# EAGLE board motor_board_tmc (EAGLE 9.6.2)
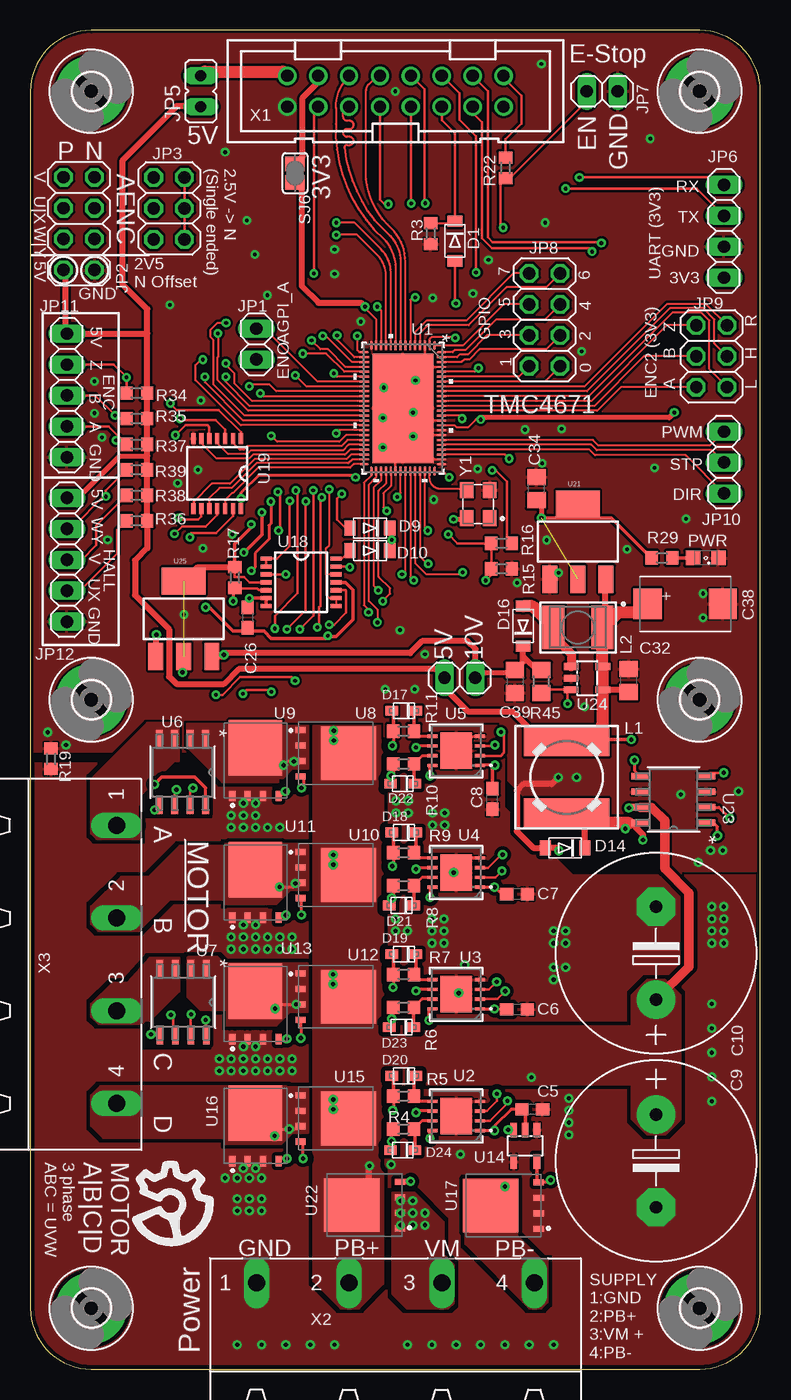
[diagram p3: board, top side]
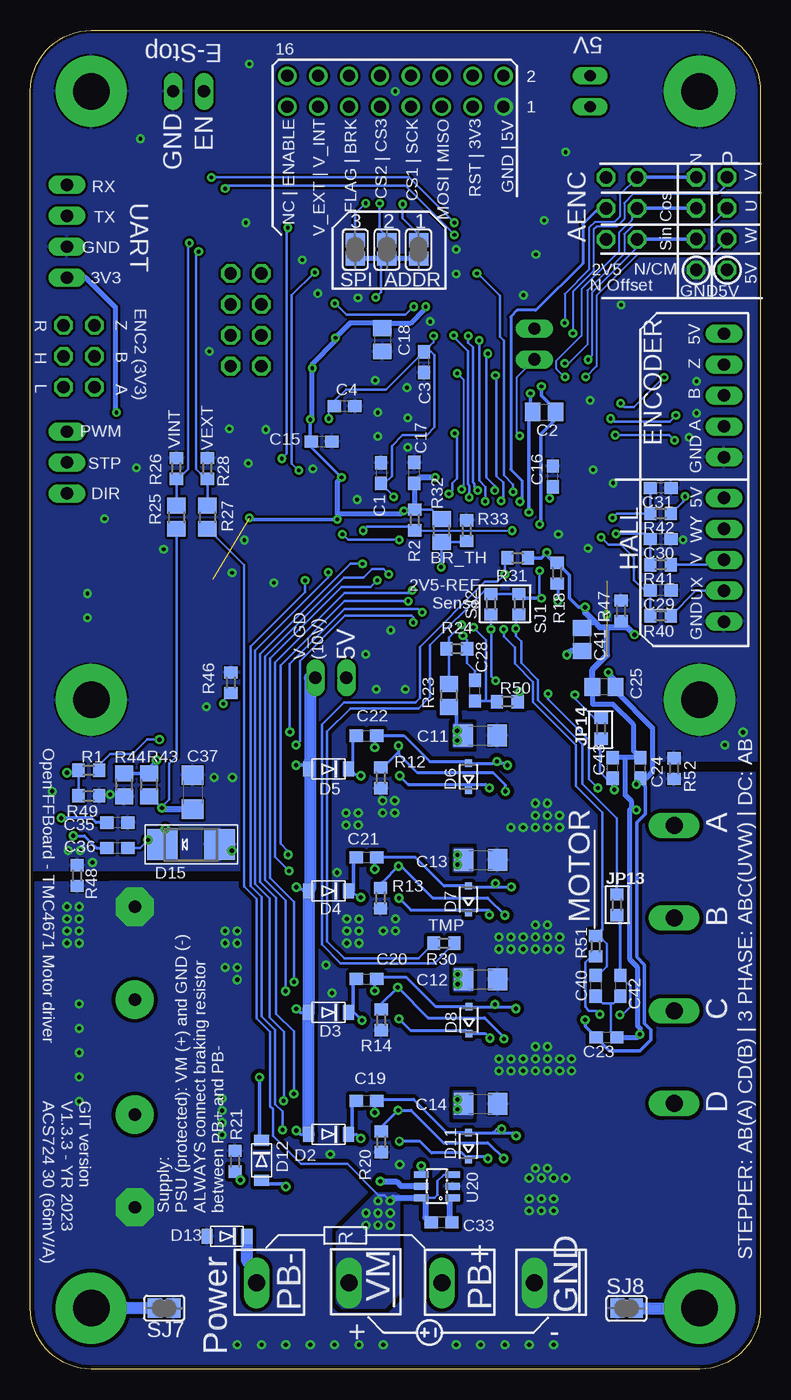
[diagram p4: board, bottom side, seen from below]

Size 60 x 110 mm. Coordinates in mm from the lower left corner, seen from the top.
Outline: 0,5 arc90 5,0 55,0 arc90 60,5 60,105 arc90 55,110 5,110 arc90 0,105 0,5
Copper layers (1*16): Top 0.07mm / dielectric 1.5mm / Bottom 0.07mm
Design rules "jlcpcb *": minimum track width 5mil, minimum drill 0.3mm, track to track 8mil, track to pad 8mil, pad to pad 8mil, via to via 8mil, smd to smd 5mil, copper to edge 0.2mm, drill to drill 8mil, minimum pad ring 10mil, minimum via ring 8mil, stop-mask expansion 4mil, vias tented up to drill 0.4mm, thermal gap 6mil

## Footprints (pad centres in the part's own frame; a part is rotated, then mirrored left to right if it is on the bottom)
C0603 = smd 1.1 x 1: 1 -0.85,0; 2 0.85,0
C0805 = smd 1.3 x 1.5: 1 -0.95,0; 2 0.95,0
E7,5-16 = drill 1.016 pad 3.15: + -3.81,0 | drill 1.016 pad 3.15 octagon: - 3.81,0
C1206 = smd 1.6 x 1.8: 1 -1.4,0; 2 1.4,0
CAPPM7343X310N = smd 2.31 x 2.52: 1 -3.1,0; 2 3.1,0
SOD-123FL = smd 0.91 x 1.22: A 1.637,0; C -1.637,0
SOD323-R = smd 0.6 x 0.6: A 1.1,0; C -1.1,0
SMADIODE = smd 2.54 x 2.54: A 2.349,0; C -2.349,0
SOD-323F = smd 1 x 0.8: A -1,0; C 1,0
3,0-PAD = drill 3 pad 5.842: B3,0 0,0
1X02 = drill 1.016 long: 1 -1.27,0; 2 1.27,0
2X04 = drill 1.016 octagon: 1 -3.81,-1.27; 2 -3.81,1.27; 3 -1.27,-1.27; 4 -1.27,1.27; 5 1.27,-1.27; 6 1.27,1.27; 7 3.81,-1.27; 8 3.81,1.27
2X03 = drill 1.016 octagon: 1 -2.54,-1.27; 2 -2.54,1.27; 3 0,-1.27; 4 0,1.27; 5 2.54,-1.27; 6 2.54,1.27
JP1 = drill 0.914 long: 1 0,-1.27; 2 0,1.27
1X04 = drill 1.016 long: 1 -3.81,0; 2 -1.27,0; 3 1.27,0; 4 3.81,0
1X03 = drill 1.016 long: 1 -2.54,0; 2 0,0; 3 2.54,0
1X05 = drill 1.016 long: 1 -5.08,0; 2 -2.54,0; 3 0,0; 4 2.54,0; 5 5.08,0
RESISTOR_R0603 = smd 1 x 1.1: 1 -0.85,0; 2 0.85,0
8MMINDUCTOR = smd 2.5 x 7: 1 -3,0; 2 3,0
L4532P = smd 1.8 x 3.6: 1 -2,0; 2 2,0
SML0805 = smd 1.2 x 1.2: A 1.05,0; C -1.05,0
R0603 = smd 1 x 1.1: 1 -0.85,0; 2 0.85,0
R0805 = smd 1.3 x 1.5: 1 -0.95,0; 2 0.95,0
SJ = smd 1.168 x 1.6: 1 -0.762,0; 2 0.762,0
QFN76_10P5X6P5 = smd 0.152 x 0.755: 1 -2.6,-5.173; 2 -2.2,-5.173; 3 -1.8,-5.173; 4 -1.4,-5.173; 5 -1,-5.173; 6 -0.6,-5.173; 7 -0.2,-5.173; 8 0.2,-5.173; 9 0.6,-5.173; 10 1,-5.173; 11 1.4,-5.173; 12 1.8,-5.173; 13 2.2,-5.173; 14 2.6,-5.173; 39 2.6,5.173; 40 2.2,5.173; 41 1.8,5.173; 42 1.4,5.173; 43 1,5.173; 44 0.6,5.173; 45 0.2,5.173; 46 -0.2,5.173; 47 -0.6,5.173; 48 -1,5.173; 49 -1.4,5.173; 50 -1.8,5.173; 51 -2.2,5.173; 52 -2.6,5.173 | smd 0.755 x 0.152: 15 3.179,-4.6; 16 3.179,-4.2; 17 3.179,-3.8; 18 3.179,-3.4; 19 3.179,-3; 20 3.179,-2.6; 21 3.179,-2.2; 22 3.179,-1.8; 23 3.179,-1.4; 24 3.179,-1; 25 3.179,-0.6; 26 3.179,-0.2; 27 3.179,0.2; 28 3.179,0.6; 29 3.179,1; 30 3.179,1.4; 31 3.179,1.8; 32 3.179,2.2; 33 3.179,2.6; 34 3.179,3; 35 3.179,3.4; 36 3.179,3.8; 37 3.179,4.2; 38 3.179,4.6; 53 -3.179,4.6; 54 -3.179,4.2; 55 -3.179,3.8; 56 -3.179,3.4; 57 -3.179,3; 58 -3.179,2.6; 59 -3.179,2.2; 60 -3.179,1.8; 61 -3.179,1.4; 62 -3.179,1; 63 -3.179,0.6; 64 -3.179,0.2; 65 -3.179,-0.2; 66 -3.179,-0.6; 67 -3.179,-1; 68 -3.179,-1.4; 69 -3.179,-1.8; 70 -3.179,-2.2; 71 -3.179,-2.6; 72 -3.179,-3; 73 -3.179,-3.4; 74 -3.179,-3.8; 75 -3.179,-4.2; 76 -3.179,-4.6 | smd 5.004 x 8.992: 77 0,0
SDC08A = smd 0.254 x 0.813: 1 -1.2,-1.943; 2 -0.4,-1.943; 3 0.4,-1.943; 4 1.2,-1.943; 5 1.2,1.943; 6 0.4,1.943; 7 -0.4,1.943; 8 -1.2,1.943 | smd 2.997 x 2.591: 9 0,0
SOIC8_D_TEX = smd 1.46 x 0.559: 1 -2.724,1.905; 2 -2.724,0.635; 3 -2.724,-0.635; 4 -2.724,-1.905; 5 2.724,-1.905; 6 2.724,-0.635; 7 2.724,0.635; 8 2.724,1.905
MOSFET_BSC093N04LSGATMA1 = smd 0.5 x 0.85: 1 -1.905,-2.9; 2 -0.635,-2.9; 3 0.635,-2.9; 4 1.905,-2.9 | smd 4.41 x 4.55: 5 0,1.05
SOT23-5L = smd 0.55 x 1.2: 1 -0.95,-1.3; 2 0,-1.3; 3 0.95,-1.3; 4 0.95,1.3; 5 -0.95,1.3
TSSOP14 = smd 0.9 x 0.35: 1 -2.875,1.95; 2 -2.875,1.3; 3 -2.875,0.65; 4 -2.875,0; 5 -2.875,-0.65; 6 -2.875,-1.3; 7 -2.875,-1.95; 8 2.875,-1.95; 9 2.875,-1.3; 10 2.875,-0.65; 11 2.875,0; 12 2.875,0.65; 13 2.875,1.3; 14 2.875,1.95
SOT23-6 = smd 0.55 x 1.2: 1 -0.95,-1.3; 2 0,-1.3; 3 0.95,-1.3; 4 0.95,1.3; 5 0,1.3; 6 -0.95,1.3
SOT223 = smd 1.219 x 2.235: 1 -2.311,-3.099; 2 0,-3.099; 3 2.311,-3.099 | smd 3.6 x 2.2: 4 0,3.099
21-0041B_8_MXM = smd 0.543 x 1.455: 1 -1.905,-2.721; 2 -0.635,-2.721; 3 0.635,-2.721; 4 1.905,-2.721; 5 1.905,2.721; 6 0.635,2.721; 7 -0.635,2.721; 8 -1.905,2.721
PAK100/2500-16 = drill 1 pad 1.422: 1 -8.89,-1.27; 2 -8.89,1.27; 3 -6.35,-1.27; 4 -6.35,1.27; 5 -3.81,-1.27; 6 -3.81,1.27; 7 -1.27,-1.27; 8 -1.27,1.27; 9 1.27,-1.27; 10 1.27,1.27; 11 3.81,-1.27; 12 3.81,1.27; 13 6.35,-1.27; 14 6.35,1.27; 15 8.89,-1.27; 16 8.89,1.27
GMSTBA4 = drill 1.397 long: 1 -11.43,5.08; 2 -3.81,5.08; 3 3.81,5.08; 4 11.43,5.08
ECS-327KE-TR = smd 1.3 x 1.1: 1 -1.15,-0.95; 2 1.15,-0.95; 3 1.15,0.95; 4 -1.15,0.95

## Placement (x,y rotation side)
C1  100nF  [C0603]  31.18,73.62 270 bottom
C2  10µF  [C0805]  17.77,78.65 0 bottom
C3  100nF  [C0603]  27.65,82.75 90 bottom
C4  100nF  [C0603]  34.17,79.12 180 bottom
C5  100nF  [C0603]  41.25,21.35 180 top
C6  100nF  [C0603]  40,29.55 180 top
C7  100nF  [C0603]  40,39.03 180 top
C8  100nF  [C0603]  37.98,46.85 90 top
C9  680µF  [E7,5-16]  51.42,17.1 270 top
C10  680µF  [E7,5-16]  51.42,34.17 90 top
C11  1µF  [C1206]  23.02,52.05 0 bottom
C12  1µF  [C1206]  22.98,32.03 0 bottom
C13  1µF  [C1206]  23,41.85 0 bottom
C14  1µF  [C1206]  23,21.8 0 bottom
C15  100nF  [C0603]  36.08,76.22 0 bottom
C16  100nF  [C0603]  17.05,73.35 90 bottom
C17  100nF  [C0603]  28.45,73.65 90 bottom
C18  10µF  [C0805]  31.07,84.58 270 bottom
C19  100nF  [C0603]  32.38,22.05 0 bottom
C20  100nF  [C0603]  32.38,32.05 0 bottom
C21  100nF  [C0603]  32.38,42.05 0 bottom
C22  100nF  [C0603]  32.38,52.05 0 bottom
C23  100nF  [C0603]  12.65,27.25 180 bottom
C24  100nF  [C0603]  9.88,49.4 90 bottom
C25  10µF  [C0805]  12.85,56.05 180 bottom
C26  100nF  [C0603]  17.85,61.75 270 top
C28  4.7nF  [C0603]  23.45,55.75 90 bottom
C29  4.7nF  [C0603]  8.2,64 180 bottom
C30  4.7nF  [C0603]  8.2,68.2 180 bottom
C31  4.7nF  [C0603]  8.2,72.4 180 bottom
C32  10µF  [C0805]  49.17,56.58 90 top
C33  100nF  [C0603]  26.2,12.05 180 bottom
C34  10µF  [C0805]  41.6,72.35 90 top
C35  100nF  [C0603]  52.85,44.9 180 bottom
C36  100nF  [C0603]  52.85,42.83 0 bottom
C37  1µF  [C1206]  46.67,47.4 270 bottom
C38  593D476X0016D2TE3  [CAPPM7343X310N]  53.83,62.88 0 top
C39  10µF  [C0805]  39.83,56.5 270 top
C40  4.7nF  [C0603]  13.55,31.5 270 bottom
C41  10µF  [C0805]  14.65,59.95 90 bottom
C42  100nF  [C0603]  11.5,31.5 270 bottom
C43  100nF  [C0603]  12.15,49.4 90 bottom
D1  LV low drop  [SOD-123FL]  34.9,92.7 270 top
D2  HV >100V  [SOD-123FL]  35.5,19.3 180 bottom
D3  HV >100V  [SOD-123FL]  35.5,29.3 180 bottom
D4  HV >100V  [SOD-123FL]  35.5,39.3 180 bottom
D5  HV >100V  [SOD-123FL]  35.5,49.3 180 bottom
D6  BZX384-XXX  [SOD323-R]  24,48.67 90 bottom
D7  BZX384-XXX  [SOD323-R]  24,38.6 90 bottom
D8  BZX384-XXX  [SOD323-R]  23.95,28.67 90 bottom
D9  LV low drop  [SOD-123FL]  27.9,69.1 180 top
D10  LV low drop  [SOD-123FL]  27.9,67.25 180 top
D11  BZX384-XXX  [SOD323-R]  24,18.33 90 bottom
D12  HV >100V  [SOD-123FL]  41,17.15 270 bottom
D13  Zener 65V (MMSZ5265BT1G)  [SOD-123FL]  43.85,10.9 180 bottom
D14  HV >100V  [SOD-123FL]  43.95,42.83 180 top
D15  HV >100V  [SMADIODE]  46.8,43.1 0 bottom
D16  LV low drop  [SOD-123FL]  40.5,61.05 90 top
D17  [SOD-323F]  30.7,54.1 0 top
D18  [SOD-323F]  30.7,44.1 0 top
D19  [SOD-323F]  30.7,34.1 0 top
D20  [SOD-323F]  30.7,24.1 0 top
D21  [SOD-323F]  30.5,38.1 0 top
D22  [SOD-323F]  30.6,48.1 0 top
D23  [SOD-323F]  30.5,28.1 0 top
D24  [SOD-323F]  30.6,18 0 top
H1  MOUNT-PAD-ROUND3.0  [3,0-PAD]  55,5 0 top
H2  MOUNT-PAD-ROUND3.0  [3,0-PAD]  5,5 0 top
H3  MOUNT-PAD-ROUND3.0  [3,0-PAD]  55,105 0 top
H4  MOUNT-PAD-ROUND3.0  [3,0-PAD]  55,55 0 top
H5  MOUNT-PAD-ROUND3.0  [3,0-PAD]  5,105 0 top
H6  MOUNT-PAD-ROUND3.0  [3,0-PAD]  5,55 0 top
JP1  [1X02]  18.57,84.22 90 top
JP2  [2X04]  4,94.12 90 top
JP3  [2X03]  11.4,95.38 270 top
JP4  V_DRV  [1X02]  35.3,56.8 180 top
JP5  [JP1]  14,105 0 top
JP6  [1X04]  57,93.5 270 top
JP7  [1X02]  47,105 180 top
JP8  [2X04]  42.27,86.22 90 top
JP9  [2X03]  56,83.22 90 top
JP10  [1X03]  57,74.5 270 top
JP11  [1X05]  3,80 270 top
JP12  [1X05]  3,66.5 270 top
JP13  JUMPER-SMT_2_NO_SILK  [RESISTOR_R0603]  11.8,38.15 90 bottom
JP14  JUMPER-SMT_2_NO_SILK  [RESISTOR_R0603]  13.1,52.65 90 bottom
L1  220µH  [8MMINDUCTOR]  44.08,48.62 90 top
L2  10µH  [L4532P]  45,60.95 180 top
LED1  Green  [SML0805]  55.5,66.65 180 top
R1  47k  [R0603]  55.2,49.2 0 bottom
R2  10k  [R0603]  28.4,69.78 90 bottom
R3  10k  [R0603]  32.9,93.3 90 top
R4  10  [R0603]  30.68,19.72 0 top
R5  10  [R0603]  30.68,22.42 0 top
R6  10  [R0603]  30.68,29.72 0 top
R7  10  [R0603]  30.68,32.42 0 top
R8  10  [R0603]  30.68,39.72 0 top
R9  10  [R0603]  30.68,42.42 0 top
R10  10  [R0603]  30.68,49.73 0 top
R11  10  [R0603]  30.68,52.42 0 top
R12  36k  [R0603]  31.2,48.58 90 bottom
R13  36k  [R0603]  31.23,38.7 90 bottom
R14  36k  [R0603]  31.18,28.7 90 bottom
R15  10k  [R0603]  38.73,65.75 180 top
R16  1.5k  [R0603]  38.73,67.85 180 top
R17  10k  [R0603]  16.8,65.05 90 top
R18  10k  [R0603]  16.7,65.4 270 bottom
R19  0  [R0603]  1.7,50.15 270 top
R20  36k  [R0603]  31.15,18.67 90 bottom
R21  36k  [R0603]  43.17,17.08 270 bottom
R22  1.5k  [R0603]  39.05,98.7 90 top
R23  71.5k  [R0805]  25.6,55.35 270 bottom
R24  1.5k  [R0603]  24.95,59.2 180 bottom
R25  294k  [R0805]  48,70 270 bottom
R26  10k  [R0603]  48,74 270 bottom
R27  294k  [R0805]  45.45,70 270 bottom
R28  10k  [R0603]  45.45,74 270 bottom
R29  1.5k  [R0603]  51.9,66.65 180 top
R30  10k thermistor  [R0603]  26,35 180 bottom
R31  1.5k  [R0603]  19.95,66.65 180 bottom
R32  71.5k  [R0805]  26.2,68.9 90 bottom
R33  47k  [R0603]  24.15,68.9 270 bottom
R34  4.7k  [R0603]  8.75,80.2 0 top
R35  4.7k  [R0603]  8.75,78.1 0 top
R36  4.7k  [R0603]  8.75,69.7 0 top
R37  4.7k  [R0603]  8.75,76 0 top
R38  4.7k  [R0603]  8.75,71.8 0 top
R39  4.7k  [R0603]  8.75,73.9 0 top
R40  1.5k  [R0603]  8.2,61.9 0 bottom
R41  1.5k  [R0603]  8.2,66.1 0 bottom
R42  1.5k  [R0603]  8.2,70.3 0 bottom
R43  294k  [R0805]  50.25,48 270 bottom
R44  71.5k  [R0805]  52.3,48 270 bottom
R45  71.5k  [R0805]  42,56.5 90 top
R46  10k  [R0603]  43.52,56.4 270 bottom
R47  0  [R0603]  11.45,62.3 90 bottom
R48  0  [R0603]  56.15,40.55 270 bottom
R49  15k  [R0603]  55.2,47.1 180 bottom
R50  1.5k  [R0603]  20.8,54.85 0 bottom
R51  1.5k  [R0603]  13.55,34.75 270 bottom
R52  0  [R0603]  7.1,49.35 270 bottom
SJ1  0R  [RESISTOR_R0603]  22.15,62.85 270 bottom
SJ2  0R  [RESISTOR_R0603]  19.85,62.85 270 bottom
SJ3  [SJ]  28.1,92 270 bottom
SJ4  [SJ]  30.7,92 270 bottom
SJ5  [SJ]  33.3,92 270 bottom
SJ6  3.3V  [SJ]  21.75,98.28 270 top
SJ7  [SJ]  49,5 180 bottom
SJ8  [SJ]  11,5 0 bottom
U1  TMC4671  [QFN76_10P5X6P5]  30.62,78.95 180 top
U2  LM5109BSD  [SDC08A]  35,20.8 90 top
U3  LM5109BSD  [SDC08A]  35,30.8 90 top
U4  LM5109BSD  [SDC08A]  35,40.8 90 top
U5  LM5109BSD  [SDC08A]  35,50.8 90 top
U6  TMCS1100  [SOIC8_D_TEX]  12.5,49.05 270 top
U7  TMCS1100  [SOIC8_D_TEX]  12.55,30.15 270 top
U8  BSC030N08NS5ATMA1  [MOSFET_BSC093N04LSGATMA1]  25.1,50.6 270 top
U9  BSC030N08NS5ATMA1  [MOSFET_BSC093N04LSGATMA1]  18.5,50 0 top
U10  BSC030N08NS5ATMA1  [MOSFET_BSC093N04LSGATMA1]  25.1,40.6 270 top
U11  BSC030N08NS5ATMA1  [MOSFET_BSC093N04LSGATMA1]  18.5,40 0 top
U12  BSC030N08NS5ATMA1  [MOSFET_BSC093N04LSGATMA1]  25.1,30.6 270 top
U13  BSC030N08NS5ATMA1  [MOSFET_BSC093N04LSGATMA1]  18.5,30 0 top
U14  MCP14XX  [SOT23-5L]  40.67,18.35 180 top
U15  BSC030N08NS5ATMA1  [MOSFET_BSC093N04LSGATMA1]  25.1,20.6 270 top
U16  BSC030N08NS5ATMA1  [MOSFET_BSC093N04LSGATMA1]  18.5,20 0 top
U17  BSC030N08NS5ATMA1  [MOSFET_BSC093N04LSGATMA1]  38.88,13.42 90 top
U18  MCP6004  [TSSOP14]  22.25,64.65 0 top
U19  74LV17APWJ  [TSSOP14]  15.35,73.6 270 top
U20  LM74700-Q1  [SOT23-6]  26.57,15.03 90 bottom
U21  [SOT223]  45,68 0 top
U22  BSC030N08NS5ATMA1  [MOSFET_BSC093N04LSGATMA1]  27.48,13.47 90 top
U23  MAX5033BASA+T  [21-0041B_8_MXM]  52.85,46.8 90 top
U24  AP3012KTR-G1  [SOT23-5L]  45.75,56.77 270 top
U25  [SOT223]  12.6,61.65 0 top
X1  2516-  [PAK100/2500-16]  30,105 0 top
X2  GMSTBA4  [GMSTBA4]  30,2 0 top
X3  GMSTBA4  [GMSTBA4]  2,33.25 270 top
Y1  25MHz  [ECS-327KE-TR]  36.8,71.08 90 top

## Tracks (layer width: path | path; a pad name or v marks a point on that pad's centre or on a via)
2.5V_REF  (via drill 0.3)
  Top 0.2: JP3.2 JP3.4 JP3.6
  Top 0.254: v18.15,65.6 18.47,65.92 18.47,67.05 19.62,68.19 19.62,69.33 19.77,69.48 v19.77,71.28
  Top 0.3: C26.1 17.85,63.2 v18,63.35
  Top 0.305: U18.7 U18.6 v18,63.35
  Bottom 0.2: 19.85,63.35 SJ2.1 SJ1.1 22.36,63.91 22.72,63.91 27.15,59.48 27.15,55.25 28.1,54.3 33.7,54.3 35.6,52.4 35.6,35.15 34.2,33.75 28.1,33.75 R30.2 | v18.15,65.6 18.15,63.5 v18,63.35
  Bottom 0.254: JP3.4 12.82,95.53 13.16,95.53 14.61,94.08 14.61,90.85 18.46,87 20,87 20.52,86.48 20.52,73.92 19.62,73.01 19.62,71.43 v19.77,71.28
  Bottom 0.305: 19.85,63.35 v18,63.35
2.5V_REF_A  (via drill 0.3)
  Top 0.152: U1.17 26.44,82.75 24.29,84.9 v24.02,84.9
  Top 0.2: v23.24,72.2 23.29,72.15 23.29,61.94 v22.15,60.8 | v15.25,55.4 15.79,55.4 17.25,56.86 21.45,56.86 v21.75,56.56
  Bottom 0.2: v24.02,84.9 24.02,84.34 23.64,83.96 23.64,72.89 23.49,72.74 23.49,72.46 v23.24,72.2 | SJ1.2 v22.15,60.8 22.09,60.74 22.09,56.9 v21.75,56.56 | v15.25,55.4 15.25,55.1 13.65,53.5 JP14.2
2.5V_REF_C  (via drill 0.3)
  Top 0.152: U1.19 25.8,81.95 24.3,83.44 v22.4,83.44
  Top 0.2: v21.82,72.19 21.97,72.05 21.97,63.77 20.1,61.9 v20.1,60.85
  Bottom 0.2: v22.4,83.44 22.54,83.31 22.54,73.25 21.82,72.54 v21.82,72.19 | SJ2.2 20.1,61.75 v20.1,60.85 20.1,60.25 19.65,59.8 19.65,58 18.27,56.62 18.27,54.98 14.63,51.34 14.63,48.07 11.8,45.24 JP13.2
2.5V_REF_RAW  (via drill 0.35)
  Top 0.2: R17.1 16.85,64.15 18.62,64.15 18.77,64 U18.5
  Top 0.25: R17.1 16.65,64.05 v16.65,63.1
  Bottom 0.25: R18.2 16.65,64.5 v16.65,63.1
5V_SENSE  (via drill 0.3, 0.35)  (1 unrouted)
  Top 0.152: U1.23 20.2,80.35 19.65,80.9 18.15,80.9 v18,80.75
  Top 0.2: U18.4 18.02,64.65 17.57,65.1 16.8,65.1 R17.2 16.7,65.8
  Top 0.254: 14.4,47.75 14.4,47.74 U6.8 | v14.4,28.7 14.46,28.64 U7.8
  Top 0.3: 14.4,47.75 13.5,48.65 10.8,48.65 v10.2,48.05 | 13.25,64.75 U25.4 | R17.2 16.8,67.8 18.14,69.15 v18.14,69.41
  Top 0.5: U25.2 12.5,58.45 v12.5,57.25 | U25.4 13.75,65.9 R17.2
  Bottom 0.2: v18.14,69.41 18.03,69.29 | v10.2,48.05 10.2,48.23 C24.1
  Bottom 0.3: v14.4,28.7 14.4,28.15 C23.2 12.4,26.15 9.9,26.15 9,27.05 9,27.88 9.53,28.41 9.53,33.23 10.17,33.87 10.17,44.92 9.47,45.62 9.47,47.88 9.88,48.29 C24.1 | v18,80.75 18,79.97 16.82,78.8 C2.2 16.82,78.05 18.03,76.85 18.03,69.29
  Bottom 0.4: C24.1 9.43,48.55 8.85,49.12 8.85,52.65 11.9,55.7 C25.1 11.45,56.5
  Bottom 0.5: v12.5,57.25 12.5,57.1 11.9,56.5 C25.1
+3V3  (via drill 0.3)  (1 unrouted)
  Top 0.152: U1.52 33.25,73.75 33.95,73.75 v34.42,73.28 | U1.43 29.62,72.58 29.02,71.98 29.02,70.81 v29.3,70.53 | U1.13 28.42,86.28 27.5,87.19 v27.5,87.3 | v34.92,84.75 34.92,84.8 33,84.8 32.82,84.62 U1.2 | v36.83,82.25 36.52,81.95 U1.72 | v37,78.03 36.6,78.03 35.99,77.42 35,77.42 34.87,77.55 U1.61
  Top 0.2: v17.32,71.56 17.32,70.75 U19.14
  Top 0.254: v26.73,73.28 26.57,73.42 18.74,73.42 17.32,72 v17.32,71.56
  Top 0.3: v42,69.95 45,69.95 | R29.2 47.75,69.95 45,69.95 | U21.4 45,69.95
  Top 0.4: Y1.4 35.75,69.83 v34.77,69.83 | v52.92,78.6 52.5,78.17 37.15,78.17 v37,78.03 | C34.1 42,71 v42,69.95
  Top 0.5: v27.5,87.3 27.18,87.62 23.68,87.62 22.3,89 22.3,96.96 SJ6.2
  Bottom 0.2: v29.3,70.53 29.2,70.62 R2.2 26.98,70.62 R32.2 | C15.1 37,76.3 | v17.32,71.56 17.32,72.23 C16.1
  Bottom 0.254: v34.42,73.28 36.92,75.78 C15.1
  Bottom 0.3: v27.5,87.3 27.6,87.2 | 36.91,78.12 v37,78.03 37,76.3 | v42,69.95 41.88,69.83 v34.77,69.83
  Bottom 0.4: 34.77,70.28 v34.77,69.83 | 27.6,87.2 27.6,87.1 28.77,85.92 31.07,85.92 | 36.91,78.12 36.91,82.17 v36.83,82.25 36.83,82.6 34.92,84.5 v34.92,84.75 33.73,85.95 31.07,85.95 31.07,85.92 | C17.1 28.45,71 28.93,70.53 v29.3,70.53 29.55,70.28 34.77,70.28 | v52.92,78.6 53,78.67 53,87.22 55.47,89.69 JP6.4 | C18.1 31.07,85.92 | 34.77,70.28 34.77,72.92 v34.42,73.28
  Bottom 0.5: v26.73,73.28 27.98,73.28 C17.1
+5V  (via drill 0.35)
  Top 0.2: 47.21,61.16 L2.1
  Top 0.254: C38.1 50.02,62.17 50,62.17
  Top 0.3: v49.4,51.73 46.73,51.73 46.62,51.62
  Top 0.4: JP12.1 3.88,71.58 7.33,75.03 9.6,75.03
  Top 0.5: 9.6,85.1 9.58,85.08 JP11.1 2.88,85.2 2.88,90.17 JP2.2 | 9.6,85.1 R34.2 R35.2 R37.2 9.6,75.03 R39.2 R38.2 R36.2 9.6,67.45 8.6,66.45 8.6,63.6 11.4,60.8 11.4,56.9 12,56.3 15.9,56.3 17.11,57.51 33.32,57.51 JP4.2 34.33,56.5 34.33,55.67 35.95,54.05 39.6,54.05 42.02,51.62 L1.2 45.62,51.62 47,53 | 9.6,85.1 9.6,87.1 7.6,89.1 7.6,99.35 12.03,103.78 13.95,103.78 JP5.1 | 47,55.77 U24.4 48.98,55.83 C32.1 | 47,52 46.62,51.62 | U21.3 47.21,64.8 47.21,61.16
  Top 0.8: U24.5 47,57.77
  Top 1: C38.1 51.26,63.41 | U24.4 U24.5 | 47,55.77 47,53 47,52 | 47,57.77 L2.1 47.1,60.95 48.33,62.17 50,62.17 51,62.17 51,63
  Bottom 0.2: v49.4,51.73 50.4,51.73 51.58,50.55 53.45,50.55 54.2,49.8 54.2,49.35 R1.2
AENC_UX  (via drill 0.3)
  Top 0.15: 18.2,79.55 16.75,81 16.75,81.83 16.07,82.5 v16.07,82.65
  Top 0.152: U1.25 18.2,79.55
  Bottom 0.15: 14.22,88.62 14.22,84.17 15.75,82.65 v16.07,82.65
  Bottom 0.152: 10.41,94.05 11.19,93.27 11.19,91.66 14.22,88.62 | JP2.6 2.73,95.34
  Bottom 0.2: 10.41,94.05 4.02,94.05 2.73,95.34
AENC_UX_N  (via drill 0.3)
  Top 0.15: U1.26 18.02,79.15 16.05,81.12 v16.05,81.53
  Bottom 0.152: v16.05,81.53 16.1,81.53 16.75,82.17 16.75,82.87 14.7,84.92 14.7,88.72 11.61,91.81 11.61,93.39 10.58,94.43 10.58,94.93 JP3.3 10.11,95.39
  Bottom 0.3: JP2.5 10.11,95.39
AENC_VN  (via drill 0.3)
  Top 0.15: U1.27 17.91,78.75
  Top 0.152: 17.91,78.75 15.39,81.27 15.39,83.14 15.41,83.16 v15.41,85.11
  Bottom 0.152: 10.43,96.6 11.2,95.83 11.2,94.47 11.78,93.89 13.46,93.89 13.72,93.62 13.72,90.2 15.41,88.52 v15.41,85.11
  Bottom 0.2: 2.72,97.38 3.5,96.6 10.43,96.6 | JP2.8 2.72,97.92
  Bottom 0.3: 2.72,97.92 2.72,97.38
AENC_VN_N  (via drill 0.3)
  Top 0.15: U1.28 17.62,78.35 15.04,80.94
  Top 0.152: v16.08,85.96 15.36,85.96 14.78,85.37 14.78,84.84 15.04,84.58 15.04,80.94
  Bottom 0.152: v16.08,85.96 16.08,88.35 14.08,90.35 14.08,93.77 13.61,94.25 12.01,94.25 11.56,94.7 11.56,96.49 JP3.1 10.11,97.94
  Bottom 0.3: JP2.7 10.11,97.94
AENC_WY  (via drill 0.3)
  Top 0.15: U1.29 17.48,77.95 14.35,81.08 v14.35,81.53
  Bottom 0.152: 10.03,91.67 13.47,88.22 13.47,82.4 v14.35,81.53 | JP2.4 2.73,92.8
  Bottom 0.2: 10.03,91.67 3.85,91.67 2.73,92.8
AENC_WY_N  (via drill 0.3)
  Top 0.15: U1.30 17.28,77.55 13.57,81.26 13.57,82.5
  Top 0.152: 13.57,82.5 14.03,82.95 v14.17,82.95
  Bottom 0.152: v14.17,82.95 13.83,83.29 13.83,88.47 10.13,92.17 JP3.5 10.11,92.86
  Bottom 0.3: JP2.3 10.11,92.86
AGPI_A
  Top 0.152: U1.21 23.6,81.15 19.25,85.5 JP1.2
AGPI_B  (via drill 0.3)
  Top 0.152: U1.22 22.68,80.75 v21.78,81.65
  Top 0.2: U18.2 U18.1 20.27,66.6 21.32,67.64 v21.32,71.35
  Bottom 0.2: v21.78,81.65 21.68,81.55 21.68,73.4 21.12,72.84 21.12,71.55 v21.32,71.35
BRAKE_CTRL  (via drill 0.3, 0.35)
  Top 0.2: D10.C 29.69,67.4 v29.69,68.15 29.69,69.12 29.56,69.12 D9.C | v34.35,68.6 35.1,67.85 R16.2 R15.2 37.88,65.25 v37.42,64.8
  Top 0.254: U14.3 v39.27,19.65
  Bottom 0.2: v37.42,64.8 37.42,63.85 41.92,59.36 41.92,39.71 41,38.79 41,29 39.88,27.88 39.88,21.77 39.27,21.16 v39.27,19.65 | v34.35,68.6 33.9,68.15 v29.69,68.15
BRAKE_CTRL_EXT  (via drill 0.3)
  Top 0.2: X1.12 35.25,104.83 35.25,102.65 36.6,101.3 36.6,90.15 v36.62,90.12 | R16.1 39.17,68.25 39.17,72.92 38.25,73.85 v37.95,73.85
  Bottom 0.2: v36.62,90.12 38.52,88.23 38.52,74.42 v37.95,73.85
BRAKE_CTRL_TMC  (via drill 0.3)
  Top 0.152: U1.31 25.38,77.15 v25.12,76.9
  Top 0.2: v25.6,71.92 25.2,71.53 25.2,69.8 25.9,69.1 D9.A
  Bottom 0.2: v25.12,76.9 24.95,76.72 24.95,73.17 25.3,72.83 25.3,72.22 v25.6,71.92
BRAKE_GATE  (via drill 0.35)
  Top 0.254: v42.75,15.53 42.55,15.33 U17.4
  Top 0.3: U17.4 41.65,15.45 41.65,17.03 U14.5
  Bottom 0.2: R21.2 42.75,16.22 v42.75,15.53
BRAKE_RES_COMP
  Top 0.152: D10.A 25.61,66.6 U18.14
BRAKE_RES_TH  (via drill 0.3)
  Top 0.2: U18.13 26.2,65.95 v26.25,65.9
  Bottom 0.2: R33.2 24.25,67.95 R32.1 26.2,65.95 v26.25,65.9
C_HS_A  (via drill 0.3, 0.35)
  Top 0.152: U1.39 28.02,73.43 27.42,72.83 27.42,62.77 27.79,62.4 v27.79,62.2
  Top 0.2: U5.2 38.67,50.4 38.92,50.65 38.92,52.1 v38.67,52.35
  Bottom 0.2: v38.67,52.35 38.7,52.38 38.7,57.94 34.2,62.45 28.12,62.45 27.87,62.2 v27.79,62.2
C_HS_B  (via drill 0.3, 0.35)
  Top 0.152: U1.41 28.82,73.03 28.22,72.43 28.22,64.38 v28.6,64
  Top 0.2: U4.2 38.23,40.4 v38.75,40.92
  Bottom 0.2: v38.75,40.92 39.9,42.08 39.9,58.08 34.2,63.77 28.82,63.77 v28.6,64
C_HS_C  (via drill 0.3, 0.35)
  Top 0.152: U1.46 30.8,73.75 30.8,65.55 v30.55,65.3
  Top 0.2: U3.2 38.38,30.4 v39.02,31.05
  Bottom 0.2: v39.02,31.05 39.02,38.53 40.71,40.21 40.71,58.54 34.21,65.03 32.64,65.03 31.92,65.75 31,65.75 v30.55,65.3
C_HS_D  (via drill 0.3, 0.35)
  Top 0.152: v35.52,65.47 35.35,65.3 32.55,65.3 31.62,66.23 U1.48
  Top 0.2: U2.2 37.77,20.4 39.2,21.83 v39.2,22.05
  Bottom 0.2: v39.2,22.05 39.15,22.1 39.15,27.72 40.33,28.9 40.33,38.69 41.51,39.87 41.51,59.06 35.52,65.05 v35.52,65.47
C_LS_A  (via drill 0.3, 0.35)
  Top 0.152: U1.40 28.42,73.28 27.82,72.68 27.82,63.1 28.52,62.4 v28.52,61.35
  Top 0.2: U5.3 38.1,51.2 v38.17,51.27
  Bottom 0.2: v38.17,51.27 37.85,51.6 37.85,58.2 34.12,61.92 28.68,61.92 28.52,61.77 v28.52,61.35
C_LS_B  (via drill 0.3, 0.35)
  Top 0.152: U1.42 29.22,72.78 28.62,72.18 28.62,65.1 29.56,64.16 29.56,63.71 v28.95,63.11
  Top 0.2: U4.3 37.62,41.2 38.7,42.28 v38.83,42.28
  Bottom 0.2: v38.83,42.28 38.83,42.55 39.45,43.17 39.45,57.83 34.17,63.11 v28.95,63.11
C_LS_C  (via drill 0.3, 0.35)
  Top 0.152: U1.47 31.22,65.09 v31.5,64.81
  Top 0.2: U3.3 37.7,31.2 v38.33,31.83
  Bottom 0.2: v38.33,31.83 38.33,38.4 40.3,40.37 40.3,58.37 34.42,64.26 32.05,64.26 v31.5,64.81
C_LS_D  (via drill 0.3, 0.35)
  Top 0.152: U1.49 32,73.76 32,66.75 32.58,66.17 v32.7,66.17
  Top 0.2: v38.35,22.62 38.35,22.03 37.52,21.2 U2.3
  Bottom 0.2: v38.35,22.62 38.35,27.75 39.8,29.2 39.8,38.73 41.11,40.04 41.11,58.77 33.7,66.17 v32.7,66.17
CLK_25M
  Top 0.152: Y1.3 35.75,72.33 33.7,72.33 arc-90 32.82,73.21 U1.51
CS1  (via drill 0.3)
  Top 0.2: X1.7 28.73,96.09 29.1,95.72 v29.4,95.72
  Bottom 0.2: SJ3.1 28.1,93.26 29.4,94.56 v29.4,95.72
CS2  (via drill 0.3)
  Top 0.2: X1.9 31.27,95.81 v31.3,95.78
  Bottom 0.2: v31.3,95.78 31.3,93.68 30.7,93.08 SJ4.1
CS3  (via drill 0.3)
  Top 0.2: X1.10 32.38,105.17 32.38,95.78 32.42,95.78 v32.45,95.8
  Bottom 0.2: SJ5.1 33.3,94.95 v32.45,95.8
CS_TMC  (via drill 0.3)
  Top 0.152: 31.43,88.08 31.22,87.87 U1.6
  Top 0.2: v31.62,88.08 31.43,88.08
  Bottom 0.2: v31.62,88.08 31.2,88.5 31.2,90.74 SJ4.2
  Bottom 0.4: SJ3.2 SJ4.2 SJ5.2
DIR
  Top 0.152: JP10.3 53.86,75.1 46.4,75.1 45.95,75.55 U1.56
ENABLE  (via drill 0.3)
  Top 0.152: 39.02,75.15 U1.55
  Top 0.2: v39.35,74.82 39.02,75.15 | v38.85,93.79 38.62,94.02 38.62,97.42 R22.1 39.4,97.85 45.73,104.18 JP7.2
  Bottom 0.2: v38.85,93.79 38.95,93.69 38.95,75.22 v39.35,74.82
ENC2_A
  Top 0.152: JP9.2 48.53,80.69 46.59,78.75 U1.64
ENC2_B
  Top 0.152: JP9.4 50.43,83.22 46.35,79.15 U1.65
ENC2_Z
  Top 0.152: JP9.6 52.33,85.77 46.12,79.55 U1.66
ENC_A
  Top 0.152: U1.35 26.26,75.55 25.85,75.14 18.29,75.14 17.98,74.83 15.31,74.83 14.05,76.09 U19.6
ENC_A_5V  (via drill 0.3)
  Top 0.152: v7.05,76.33 7.58,76.33 R37.1
  Top 0.2: R37.1 6.44,77.46 JP11.4 | U19.5 14.7,77.41 14.55,77.56 12.77,77.56 11.95,76.75 v11.93,76.75
  Bottom 0.2: v7.05,76.33 7.47,76.75 v11.93,76.75
ENC_B
  Top 0.152: U1.34 26.16,75.95 25.7,75.49 18.1,75.49 17.8,75.19 16.25,75.19 15.35,76.09 U19.4
ENC_B_5V  (via drill 0.3)
  Top 0.2: R35.1 7.22,78.1 v6.95,78.38 5.33,80 JP11.3 | U19.3 16,77.18 15.21,77.97 12.3,77.97 v12.3,78.1
  Bottom 0.2: v6.95,78.38 7.45,77.88 12.07,77.88 v12.3,78.1
ENC_Z
  Top 0.152: U1.33 26.05,76.35 25.55,75.85 17.83,75.85 17.52,75.55 17.2,75.55 16.65,76.09 U19.2
ENC_Z_5V  (via drill 0.3)
  Top 0.2: JP11.2 6.86,82.54 v7.9,81.5 R34.1 | U19.1 17.3,77 15.48,78.82 12.03,78.82 v11.5,79.35
  Bottom 0.2: v11.5,79.35 11.2,79.05 10.4,79.05 7.92,81.53 v7.9,81.5
ENO  (via drill 0.3)
  Top 0.152: U1.32 25.95,76.75 25.41,76.21 20.28,76.21 v19.79,76.7
  Bottom 0.152: JP1.1 20.05,81.48 20.05,76.96 v19.79,76.7
FLAG
  Top 0.152: R3.2 34.85,94.15 34.9,94.2 D1.C
  Top 0.2: X1.11 33.81,102.63 34.9,101.54 D1.C
G_HS_A  (via drill 0.35)
  Top 0.254: v22.27,47.75 22.48,47.75 22.48,48.42 U8.4 | R10.1 29.82,48.92 v29.65,48.75
  Top 0.3: D22.A 29.6,48.7 v29.65,48.75
  Bottom 0.2: D6.C 24,48.05
  Bottom 0.254: v22.27,47.75 22.57,48.05 24,48.05 28.95,48.05 v29.65,48.75
G_HS_B  (via drill 0.35)
  Top 0.254: v22.27,37.33 22.27,38.62 U10.4 | R8.1 29.82,38.83 v29.7,38.7
  Top 0.3: D21.A 29.5,38.5 v29.7,38.7
  Bottom 0.2: D7.C 24,37.72
  Bottom 0.254: 24,37.72 22.27,37.72 v22.27,37.33 | v29.7,38.7 28.73,37.72 24.23,37.72 D7.C
G_HS_C  (via drill 0.35)
  Top 0.254: U12.4 22.2,28.1 22.23,28.08 v22.23,27.2 | v29.7,28.78 29.82,28.9 R6.1
  Top 0.3: D23.A 29.5,28.58 v29.7,28.78
  Bottom 0.254: v22.23,27.2 22.6,27.58 D8.C 24.23,27.85 28.77,27.85 v29.7,28.78
G_HS_D  (via drill 0.35)
  Top 0.254: v22.4,17.3 22.4,18.5 U15.4 | v29.68,18.72 29.68,19.58 R4.1
  Top 0.3: D24.A 29.68,18.08 v29.68,18.72
  Bottom 0.2: D11.C 24,17.47
  Bottom 0.254: 24,17.47 22.45,17.47 22.4,17.42 v22.4,17.3 | D11.C 24.52,17.75 27.02,17.75 28,18.72 v29.68,18.72
G_LS_A  (via drill 0.35)
  Top 0.254: U9.4 20.57,47.1 v20.95,47.48 | R11.1 29.82,51.3 v29.75,51.23
  Top 0.3: D17.A 29.82,53.98 R11.1
  Bottom 0.152: R12.2 31.02,49.42 30.73,49.73
  Bottom 0.254: v20.95,47.48 20.95,47.98 21.97,49.01 28.21,49.01 29.75,50.55 | v29.75,51.23 29.75,50.55 | 29.75,50.55 29.82,50.62 30.73,49.73
G_LS_B  (via drill 0.35)
  Top 0.254: U11.4 20.8,37.1 v21,37.3 | R9.1 29.82,41.4 v29.75,41.33
  Top 0.3: D18.A 29.82,43.97 R9.1
  Bottom 0.152: R13.2 31.04,39.74 31.04,40.04
  Bottom 0.254: v21,37.3 22.43,38.72 26.95,38.72 29.55,41.33 v29.75,41.33 31.04,40.04
G_LS_C  (via drill 0.35)
  Top 0.254: U13.4 20.43,27.12 v21.07,27.12 | R7.1 29.82,31.39 v29.8,31.37
  Top 0.3: D19.A 29.82,33.97 R7.1
  Bottom 0.152: R14.2 31.18,29.99
  Bottom 0.254: v21.07,27.12 21.07,27.28 22.68,28.88 27.31,28.88 v29.8,31.37 31.18,29.99
G_LS_D  (via drill 0.35)
  Top 0.254: v21.1,17.3 20.61,17.3 U16.4 | R5.1 29.82,21.32 v29.77,21.27
  Top 0.3: D20.A 29.82,23.97 R5.1
  Bottom 0.152: R20.2 31.15,19.89
  Bottom 0.254: v21.1,17.3 22.4,18.6 26.05,18.6 28.72,21.27 v29.77,21.27 31.15,19.89
GND  (via drill 0.3, 0.35)
  Top 0.152: 30.62,80 30.62,81.87 31.1,82.35 32.5,82.35 | 30.62,80 U1.77 | 30.62,80 30.57,79.95 29,79.95 30,78.95 U1.77 | U1.54 33.25,74.75 31.5,76.5 | 31.42,76.75 31.59,76.59 31.5,76.5 | 31.42,76.75 30.62,77.55 30.62,78 | 30.62,78 U1.77 | U1.62 32.55,77.95 32.5,78 30.62,78 | U1.73 32.5,82.35 | U1.3 32.42,82.43 32.5,82.35 | U1.44 30.02,74.98 30,75 31.5,76.5 | U1.59 31.42,76.75
  Top 0.5: v43.4,48.62 42.85,48.08 40.54,48.08 39.97,47.51 39.97,44.19 41.33,42.83 D14.A 43.23,42.83 v43.45,42.6
  other vias: 16,100 30,105 25,92 36.38,88.38 42.3,94.2 42,107.25 25,90 29.05,80.65 50.95,101.1 11.45,87.45 36.77,73.97 51.3,74.05 17.77,94.4 13.75,73.9 45.3,83.62 31.65,81.25 28.98,78.17 31.45,78.6 28.98,75.75 31.45,76.65 33.15,71.45 27.15,86.08 5.25,81.15 5.25,78.55 6.35,68.15 5.88,76.58 18.45,91.6 12.1,72.8 19.48,88.25 14.18,67.45 37.65,91.15 49.05,67.35 45.55,54.42 40,64.6 43.65,77.25 40.65,77.2 16.6,68.6 44.9,48.62 53.9,69.88 55.3,63.73 14,79.6 30.38,60.73 12.62,62 33.08,88.03 53.45,47.23 55.9,42.62 54.9,41.62 56.9,42.62 1.43,52.33 2.92,51.27 43.42,65.42 42.08,74.42 55.3,61.73 58.2,47.48 29.18,55.88 31.57,55.88 42.42,68.12 32.42,58.73
  pour Bottom (rank 6): -0.45,50 -0.45,111 60.3,111 60.3,41 42.2,41 42.2,50
  pour Top (rank 6): -0.6,50.67 -0.6,111 60.3,111 60.3,40.25 47.35,40.25 36.9,50.7
  pour Top (no thermals): 22,105 20,105 20,102.65 22,102.65
  pour Bottom (no thermals): 22,105 20,105 20,102.65 22,102.65
  cutout Top: 9,45.35 14.85,45.35 14.85,48.5 11.25,48.5 9,46.25
GND1
  cutout Top: 9.2,26.35 14.75,26.35 14.75,28.45 9.5,28.45 9.2,28.15
GNDA  (via drill 0.3, 0.35)
  Top 0.152: v18.9,80.18 19.13,79.95 U1.24
  Top 0.3: U18.11 25.89,64.65 26.53,64.01 26.53,61.59 25.13,60.19 24.5,60.19 v24.45,60.24 24.26,60.05 19.78,60.05 19.2,60.63 18,60.63 | v17.55,67.1 19.02,68.58 v19.02,70.4 | 18,60.63 16.67,60.63 14.7,62.6 v14.4,62.6 | C26.2 18,60.75 18,60.63
  Top 0.4: U7.5 10.57,27.5 v9.9,27.5 | U6.5 10.58,46.33 v10.2,45.95
  Top 0.5: v10.35,60.35 10.29,60.29 U25.1
  Bottom 0.2: 12.3,30.05 12.1,30.05 C42.2 | 12.3,30.05 12.95,30.05 C40.2 | C23.1 12.3,27.75 12.3,30.05 | C28.2 23.45,57.35 24.1,58 R24.1 24.1,59.89 v24.45,60.24
  Bottom 0.25: 23.4,56.65 C28.2
  Bottom 0.3: v18.9,80.18 18.9,78.65 C2.1 19.02,78.35 v19.02,70.4 | 10.72,46 10.57,46 10.25,46 v10.2,45.95 | R31.1 18,66.65 v17.55,67.1 17.55,66.85 16.94,66.24 16.94,66.25 R18.1 15.7,65.25 15.7,63.35 14.95,62.6 v14.4,62.6
  Bottom 0.4: C23.1 10.15,27.25 v9.9,27.5 9.9,28 10.08,28.18 10.08,33 10.72,33.64 10.72,46 | 11.11,50.25 11.11,47.16 10.57,46.62 10.57,46 | 11.11,50.25 C43.2 | 11.11,50.25 C24.2 10.41,50.79 10.41,52.91 12.15,54.65 13.8,54.65 C25.2
  Bottom 0.5: v10.35,60.35 10.95,60.95 11,60.95 | 11,60.95 12.6,60.95 | 12.6,60.95 13.2,60.95 13.62,61.38 | 13.62,61.38 14.4,62.15 v14.4,62.6 | C25.2 13.8,57.48 12.6,58.68 12.6,60.95 | R47.1 11.45,61.4 11,60.95 | C41.2 14.18,61.38 13.62,61.38
GNDI  (via drill 0.35)
  Top 0.2: U3.9 35,30.84 | U4.9 35,41.28 35.36,41.64 | U5.4 35.78,52 35,51.22 U5.9
  Top 0.3: U4.4 35.73,42 35.36,41.64
  other vias: 18.5,45.5 17.5,45.5 16.5,45.5 16.5,44.5 17.5,44.5 19.5,44.5 18.5,44.5 17.5,46.5 20.5,44.5 18.5,46.5 19.5,35.5 18.5,35.5 17.5,35.5 16.5,35.5 16.5,34.5 17.5,34.5 19.5,34.5 18.5,34.5 17.5,36.5 18.5,36.5 20.5,34.5 20.5,35.5 21.5,35.5 21.5,34.5 19.5,25.5 18.5,25.5 17.5,25.5 16.5,25.5 16.5,24.5 17.5,24.5 19.5,24.5 18.5,24.5 15.53,24.5 17.5,26.5 18.5,26.5 15.53,25.5 20.5,24.5 20.5,25.5 21.5,25.5 21.5,24.5 19,13 17,13 19,15.7 18,15.7 17,15.7 16,15.7 17.5,16.5 18.5,16.5 19,14 17,14 18,14 18,13 25,2 23,2 21,2 19,2 17,2 41,2 39,2 37,2 35,2 33,2 31,2 43,2 34.05,44.7 33.05,45.7 34.05,45.7 33.05,44.7 30.05,46.7 31.05,46.7 31.05,45.7 30.05,45.7 34,35 34,36 33,37 30,37 34,37 33,35 33,36 30,36 31,36 35.35,17.65 29.65,16.8 44,36 44,35 44,33 43,32 43,33 43,35 43,36 44.25,19.25 44.25,20.25 44.25,21.25 44.25,22.25 56,36 57,36 57,35 56,35 56,38 57,38 57,37 56,37 56,30 56,28 56,26 56,24 56,22 35.7,33.2 35.2,30.9 34.8,40.8
  pour Top (no thermals): 16.15,44.5 19.5,44.5 19.5,47.7 16.15,47.7
  pour Top (no thermals): 16.15,34.5 19.5,34.5 19.5,37.8 16.15,37.8
  pour Top (no thermals): 16.15,24.5 19.5,24.5 19.5,27.7 16.15,27.7
  pour Top (no thermals): 16.15,15.5 19.5,15.5 19.5,17.7 16.15,17.7
  pour Top (no thermals): 53.42,15.1 49.42,15.1 49.42,11.1 53.42,11.1
  pour Bottom (no thermals): 53.42,15.1 49.42,15.1 49.42,11.1 53.42,11.1
  pour Bottom (no thermals): 53.45,40.03 49.45,40.03 49.45,36.03 53.45,36.03
  pour Top (isolate 0.5, no thermals): 53.45,40.03 49.45,40.03 49.45,36.03 53.45,36.03
  pour Bottom (isolate 0.305, rank 3): 0,-1 0,49 15,49 15,54.05 37,54.05 37,43 40,40 60,40 60,-1
  pour Top (isolate 0.305, rank 3): 0,-1 0,49.75 37,49.75 37,48.1 44.55,40.55 60,40.55 60,-1
  pour Top: 33,52.85 38.9,52.85 38.9,45.1 33,45.1
  pour Top (no thermals): 41,14.47 43,14.47 43,11 41,11
  pour Top (no thermals): 17,9.78 20.45,9.78 20.45,4 17,4
  pour Bottom (no thermals): 17,9.78 20.45,9.78 20.45,4 17,4
GPIO0
  Top 0.152: JP8.1 42.28,81.15 U1.70
GPIO1
  Top 0.152: JP8.2 40.14,81.55 U1.71
GPIO2
  Top 0.152: JP8.3 42.4,83.81 36.93,83.81 36.09,82.97 35.66,82.97 35.44,82.75 U1.74
GPIO3
  Top 0.152: JP8.4 37.53,84.95 35.95,83.36 35.28,83.36 35.07,83.15 U1.75
GPIO4
  Top 0.152: JP8.5 42.27,86.22 38.24,86.22 35.77,83.75 34.9,83.75 34.7,83.55 U1.76
GPIO5
  Top 0.152: JP8.6 38.93,87.5 35.55,84.12 U1.1
GPIO6
  Top 0.152: JP8.7 42.4,88.89 39.13,88.89 36.02,85.78 32.68,85.78 32.02,85.12 U1.4
GPIO7
  Top 0.152: JP8.8 39.72,90.03 35.84,86.16 32.55,86.16 31.62,85.22 U1.5
HALL_UX
  Top 0.152: U1.38 26.57,74.35 26.29,74.07 18.73,74.07 16.64,71.98 16.59,71.98 16,71.4 U19.12
HALL_UX_5V  (via drill 0.3)
  Top 0.2: U19.13 16.65,70.09 15.26,68.7 13.2,68.7 13.1,68.6 v13.1,68.35
  Bottom 0.2: R40.1 C29.2 9.55,64 10.4,64.85 10.4,66.7 11.45,67.75 12.5,67.75 v13.1,68.35
HALL_V
  Top 0.152: U1.37 26.46,74.75 26.14,74.43 18.58,74.43 16.55,72.4 15.54,72.4 14.7,71.56 U19.10
HALL_V_5V  (via drill 0.3)
  Top 0.2: U19.11 15.35,70.18 14.42,69.25 12.45,69.25 v11.85,68.65
  Bottom 0.2: R41.1 C30.2 9.5,68.65 v11.85,68.65
HALL_WY
  Top 0.152: U1.36 26.36,75.15 26,74.78 18.43,74.78 16.4,72.75 14.89,72.75 13.4,71.26 U19.8
HALL_WY_5V  (via drill 0.3)
  Top 0.2: U19.9 14.05,70.05 13.8,69.8 12.3,69.8 v12.15,69.95
  Bottom 0.2: C31.2 R42.1 11.8,70.3 v12.15,69.95
INPUT_GATE  (via drill 0.35)
  Top 0.5: v31.25,15.42 31.2,15.38 U22.4
  Bottom 0.5: U20.5 29.52,15.03 29.88,15.38 31.2,15.38 v31.25,15.42
MISO
  Top 0.152: X1.6 arc45 25.1,103.64 25.1,102.32 arc50 29.01,92.89 arc-45 30.02,90.45 U1.9
MOSI
  Top 0.152: U1.8 30.42,91.02 arc45 29.55,93.12 28.27,94.4 arc-30 25.8,100.35 arc-90 26.05,100.59 26.24,100.59 arc90 26.57,100.92 26.57,100.92 arc90 26.24,101.25 26.05,101.25 arc-90 25.71,101.58 25.71,101.58 arc-90 26.05,101.91 26.24,101.91 arc90 26.57,102.24 26.57,102.24 arc90 26.24,102.57 26.05,102.57 arc-90 25.71,102.9 25.71,103.25 X1.5
MOT_A  (via drill 0.35)
  Top 0.152: 21.69,49.97 v21.65,49.92
  Top 0.2: U8.3 21.69,49.97
  Top 0.254: v21.65,49.92 21.1,49.92 v20.8,49.62 | U5.6 31.97,51.2 31.84,51.08 v31.69,51.08
  Bottom 0.152: C22.2 31.69,51.88 v31.69,51.08
  Bottom 0.2: 22,49.75 21.82,49.92 v21.65,49.92
  Bottom 0.254: v20.8,49.62 20.93,49.75 22,49.75 23.98,49.75 D6.A 24.15,49.92 27.18,49.92 29.3,52.05 31.43,52.05 31.69,51.78 v31.69,51.08
  pour Top (isolate 0.305, no thermals): 22.8,52.9 22.8,49.3 21.5,49.3 20.75,48.55 15.85,48.55 15.85,52.9
  pour Top (isolate 0.305, no thermals): 12.9,53.02 12.9,51.1 15.75,48.25 20.35,48.25 20.35,49.45 16.77,53.02
MOT_A_OUT
  pour Top (isolate 0.305, no thermals): 5,48.48 5,44 5.45,43.55 9,43.55 9,47.1 11.85,49.95 12.18,49.95 12.18,53.08 9.6,53.08
MOT_B  (via drill 0.35)
  Top 0.152: U10.3 21.84,39.97 v21.77,39.9
  Top 0.254: v20.48,39.62 21.66,39.62 22,39.97 U10.3 | U4.6 31.97,41.2 31.84,41.08 v31.69,41.08
  Bottom 0.152: C21.2 31.69,41.88 v31.69,41.08
  Bottom 0.2: v21.77,39.9 22,39.67 22,39.62
  Bottom 0.254: v31.69,41.08 31.69,41.78 31.43,42.05 28.35,42.05 26,39.7 D7.A 23.93,39.62 22,39.62 v20.48,39.62
  pour Top (isolate 0.305, no thermals): 22.8,43.2 22.8,39.33 21.32,39.33 20.2,38.2 16.02,38.2 16.02,43.2
  pour Top (isolate 0.305, no thermals): 5,38 5,36.58 5.58,36 8.9,36 11.5,38.6 20,38.6 20,43 12.25,43 9.7,40.45 7.45,40.45
MOT_C  (via drill 0.35)
  Top 0.254: v20.1,29.62 20.44,29.97 v21.82,29.97 U12.3 | U3.6 31.97,31.2 31.84,31.08 v31.69,31.08
  Bottom 0.152: C20.2 31.69,31.88 v31.69,31.08
  Bottom 0.2: 22,29.78 21.82,29.95 v21.82,29.97
  Bottom 0.254: v20.1,29.62 20.25,29.78 22,29.78 D8.A 26.68,29.78 29.1,32.2 31.27,32.2 31.69,31.78 v31.69,31.08
  pour Top (isolate 0.305, no thermals): 22.77,33.38 22.77,29.3 21.3,29.3 20.2,28.2 16.15,28.2 16.15,33.38
  pour Top (isolate 0.305, no thermals): 12.97,33.85 15.35,33.85 15.88,33.33 16.32,33.33 16.52,33.12 17.45,33.12 17.45,29.53 13.97,29.53 12.97,30.53
MOT_C_OUT
  pour Top (isolate 0.305, no thermals): 12.22,33.78 12.22,31.03 9.55,28.35 5.6,28.35 5,28.95 5,30 6.75,31.75 7.97,31.75 9.81,33.78
MOT_D  (via drill 0.35)
  Top 0.254: v20.07,19.17 20.61,19.72 v21.27,19.72 21.95,19.72 U15.3 | U2.6 31.97,21.2 31.84,21.08 v31.69,21.08
  Bottom 0.152: C19.2 31.69,21.88 v31.69,21.08
  Bottom 0.2: 22,19.42 21.71,19.72 v21.27,19.72
  Bottom 0.254: v20.07,19.17 20.32,19.42 22,19.42 D11.A 25.75,19.42 28.5,22.17 31.3,22.17 31.69,21.78 v31.69,21.08
  pour Top (isolate 0.305, no thermals): 22.8,23.2 22.8,19.38 21.52,19.38 20.6,18.45 16.05,18.45 16.05,23.2
  pour Top (isolate 0.305, no thermals): 21,19 6,19 5,20 5,22.5 5.75,23.25 21,23.25
N$1
  Top 0.2: R36.1 7.15,68.95 7.15,67 4.11,63.96 JP12.4
  Bottom 0.2: R40.2 5.29,63.96 JP12.4
N$3
  Top 0.2: R38.1 5.4,69.3 5.4,67.7 4.2,66.5 JP12.3
  Bottom 0.2: R41.2 3.4,66.1 JP12.3
N$4  (via drill 0.3)
  Top 0.152: v28.5,87.3 28.82,86.98 U1.12
  Top 0.2: D1.A 34.9,87.65 v34.98,87.58
  Bottom 0.2: v34.98,87.58 34.04,86.64 29.16,86.64 v28.5,87.3
N$5  (via drill 0.3)
  Top 0.2: v44.15,54.67 44.15,55.52 U24.3 42.27,55.83 R45.1
  Bottom 0.2: R46.2 44.15,54.92 v44.15,54.67
N$6  (via drill 0.35)
  Top 0.2: U23.4 55.87,49 v57,49
  Bottom 0.2: R49.2 R1.1 56.25,49 v57,49
N$7
  Bottom 1: SJ7.2 H1.B3,0
N$8
  Top 0.3: LED1.A 52.77,66.65 R29.1
N$9
  Top 1: X1.2 20.76,106.62 14.35,106.62 JP5.2
N$10
  Bottom 1: SJ8.2 H2.B3,0
N$12
  Top 0.75: U24.1 44.45,58.77 43.17,60.05 43.17,60.77 L2.2
  Top 1: L2.2 41.25,62.7 40.51,62.7 D16.A
N$13
  Top 0.254: U5.5 31.52,52 R11.2
  Top 0.3: R11.2 31.52,53.92 D17.C
N$15  (via drill 0.3)
  Top 0.2: R39.1 6.2,72.2 6.2,71.9 | v6.2,71.7 6.2,71.9 | 6.2,71.9 3.34,69.04 JP12.2
  Bottom 0.2: R42.2 6.35,71.3 6.35,71.55 v6.2,71.7
N$16  (via drill 0.35)
  Top 0.2: v48.9,44.4 48.8,44.5 46.2,44.5 45.9,44.8
  Top 0.5: D14.C 45.59,45.62 L1.1 | 49.2,44.87 49.23,44.89 U23.8 49.75,44.52 50.35,43.92 v50.35,43.47
  Top 0.8: L1.1 45.95,45.62 46.7,44.87
  Top 1: 49.2,44.87 46.7,44.87
  Bottom 0.2: C36.2 51,42.83 v50.35,43.47 | D15.C 49.15,44.15
  Bottom 0.4: D15.C 49.15,42.28 v50.35,43.47
  Bottom 0.5: 49.15,44.15 v48.9,44.4
N$17
  Top 0.2: X1.16 38.89,106.11 40.35,104.65 40.35,102.35 39.05,101.05 R22.2
N$18  (via drill 0.35)
  Top 0.254: v32.85,48.75 32.85,49.6 U5.8
  Bottom 0.152: C22.1 33.33,52.05
  Bottom 0.25: v32.85,48.75 33.15,48.75 33.7,49.3 D5.C
  Bottom 0.254: 33.33,52.05 33.52,51.85 33.52,49.64 D5.C
N$19  (via drill 0.35)
  Top 0.2: U23.1 56.16,44.89
  Top 0.254: v56.48,43.83 56.48,44.58 56.16,44.89
  Bottom 0.254: v56.48,43.83 55.58,43.83 54.58,42.83 C36.1
N$20
  Top 0.5: SJ6.1 22.38,99.66 22.38,104.47 23.65,105.75 X1.4
N$21  (via drill 0.35)
  Top 0.254: v49.65,50.02 49.65,49.18 U23.5
  Bottom 0.254: v49.65,50.02 50.25,49.42 R43.1 50.45,48.75
  Bottom 0.3: R44.1 R43.1
N$24
  Bottom 0.152: C33.1 25.25,12.05
  Bottom 0.5: U20.1 25.55,14.08 25.55,12.35 25.25,12.05
N$25  (via drill 0.35)
  Top 0.2: 55.62,46.12 U23.2
  Top 0.254: U23.2 56.59,46.16 v57.48,45.28
  Bottom 0.254: C35.2 54.6,44.9 55.02,45.33 57.42,45.33 v57.48,45.28
N$27
  Top 0.254: U5.7 32.2,50.4 R10.2
  Top 0.3: R10.2 31.52,48.17 D22.C
N$28  (via drill 0.35)
  Top 0.254: U4.8 32.85,39.39 v32.85,38.75
  Bottom 0.152: C21.1 33.33,42.05
  Bottom 0.2: D4.C 33.45,39.3
  Bottom 0.254: 33.6,39.3 33.05,38.75 v32.85,38.75
  Bottom 0.3: 33.33,42.05 33.45,41.92 33.45,39.3 | 33.6,39.3 D4.C
N$29
  Top 0.254: U4.5 31.52,42 R9.2
  Top 0.3: D18.C 31.7,42.6 R9.2
N$30
  Top 0.254: U4.7 32.2,40.4 R8.2
  Top 0.3: R8.2 31.52,38.12 D21.C
N$31  (via drill 0.35)
  Top 0.254: v32.85,18.95 32.85,19.6 U2.8
  Bottom 0.152: C19.1 33.33,22.05
  Bottom 0.254: v32.85,18.95 33.2,19.3 D2.C
  Bottom 0.3: 33.33,22.05 33.55,21.83 33.55,19.3 D2.C
N$32
  Top 0.254: U2.5 31.52,22 R5.2
  Top 0.3: R5.2 31.52,23.92 D20.C
N$33
  Top 0.254: U2.7 32.2,20.4 R4.2
  Top 0.3: D24.C 31.6,19.65 R4.2
N$34  (via drill 0.35)
  Top 0.254: v32.75,28.65 32.75,29.6 U3.8
  Bottom 0.152: C20.1 33.33,32.05
  Bottom 0.254: v32.75,28.65 33.4,29.3 D3.C
  Bottom 0.3: 33.33,32.05 33.48,31.9 33.48,29.3 D3.C
N$35
  Top 0.254: U3.5 31.52,32 R7.2
  Top 0.3: D19.C 31.7,32.6 R7.2
N$36
  Top 0.254: U3.7 32.2,30.4 R6.2
  Top 0.3: R6.2 31.5,29.7 D23.C
PWM_I
  Top 0.152: JP10.1 55.86,75.9 46.7,75.9 46.25,76.35 U1.58
REF_H
  Top 0.152: JP9.3 56.23,84.27 56.23,86.24 55.31,87.16 52.57,87.16 45.76,80.35 U1.68
REF_L
  Top 0.152: JP9.1 55.8,82.15 55.8,86.16 55.16,86.81 52.76,86.81 45.9,79.95 U1.67
REF_R
  Top 0.152: JP9.5 55.52,87.52 52.31,87.52 45.54,80.75 U1.69
RES_FET  (via drill 0.35)
  Top 0.254: v39,15 37.83,13.83 U17.5
  Bottom 0.254: D12.A 41,15.22
  Bottom 0.305: 41,15.22 39.23,15.22 v39,15
  Bottom 1: D13.C 42.21,8.95 41.43,8.17 X2.4
  pour Top (isolate 0.305, no thermals): 42.5,9 42.5,5.5 42,5 41.02,5 35.75,10.28 35.75,15.58 40,15.58 40,11 42,9
RESET  (via drill 0.3)
  Top 0.152: U1.50 32.4,73.75 32.4,69.17 v32.66,68.91
  Top 0.2: X1.3 23.32,103.41 23.32,90.05 v23.3,90.03 | v20.32,72.1 20.5,72.1 20.5,68.9 v20.4,68.9
  Bottom 0.152: R2.1 28.38,68.9 v20.4,68.9
  Bottom 0.2: v32.66,68.91 32.34,69.22 28.7,69.22 R2.1 | v20.32,72.1 20.32,72.7 21.07,73.45 21.07,84.5 21.4,84.83 21.4,88.2 23.23,90.03 v23.3,90.03
SCK
  Top 0.152: U1.7 30.82,90.99 arc45 29.7,93.7 29.36,94.04 arc-45 27.57,98.34 27.57,105.04 arc-45 27.79,105.55 28.5,106.27 X1.8
SENSE_A  (via drill 0.3)
  Top 0.152: v25.2,84.95 25.2,84.59 26.64,83.15 U1.16
  Top 0.2: v23.94,71.62 23.85,71.53 23.85,62.71 23.74,62.6 23.74,61.1 v23.59,60.95
  Bottom 0.2: v25.2,84.95 25.2,84.8 24.05,83.65 24.05,72.72 23.89,72.57 23.89,72.03 23.94,71.98 v23.94,71.62 | 23,54.9 C28.1 22.56,54.9 | 22.56,54.9 21.65,54.9 R50.1 | v23.59,60.95 22.56,59.92 22.56,54.9
SENSE_A_RAW  (via drill 0.3, 0.35)
  Top 0.2: U6.7 13.13,47.53 v13.35,47.75 | v17.45,55.5 17.75,55.8 19.64,55.8 v19.8,55.64
  Bottom 0.2: 13.5,47.9 v13.35,47.75 14.1,48.5 14.1,51.7 17.45,55.05 v17.45,55.5 | R50.2 19.8,55 v19.8,55.64
SENSE_C  (via drill 0.3)
  Top 0.152: U1.18 25.9,82.35 24.45,83.8 23.84,83.8 v23.11,84.53
  Top 0.2: v21.09,60.8 22.63,62.34 v22.63,71.3
  Bottom 0.2: v22.63,71.3 22.58,71.35 22.58,72.47 23.11,73 v23.11,84.53 | C40.1 13.35,32.35 12.6,33.1 12.6,34.95 13.25,35.6 R51.1 13.03,36.12 13,36.1 13,45.75 15.15,47.9 15.15,51.28 18.68,54.81 18.68,56.46 20.19,57.97 20.19,59.3 21.09,60.2 v21.09,60.8
SENSE_C_RAW  (via drill 0.35)
  Top 0.2: v13.2,29.15 13.19,29.14 U7.7
  Bottom 0.2: v13.2,29.15 13.5,29.45 14.1,29.45 14.4,29.75 14.4,33.4 13.9,33.9 R51.2
STEP
  Top 0.152: JP10.2 56,75.5 46.55,75.5 46.1,75.95 U1.57
TH_FET  (via drill 0.3)
  Top 0.2: U18.3 v21,65.3
  Bottom 0.2: R30.1 26.8,33.35 34.5,33.35 36.05,34.9 36.05,52.95 34.24,54.76 28.36,54.76 28,55.13 28,59.35 22.65,64.7 21.6,64.7 v21,65.3 21,66.45 R31.2
UART_RX  (via drill 0.3)
  Top 0.152: U1.10 29.62,90.12 arc45 28.84,92.01 26.65,94.2 v25.15,94.2
  Top 0.2: JP6.1 56.38,97.92 v45.12,97.92
  Bottom 0.2: v25.15,94.2 28.88,97.92 v45.12,97.92
UART_TX  (via drill 0.3)
  Top 0.152: U1.11 29.22,89.89 arc45 28.55,91.5 26.85,93.2 v25.15,93.2
  Top 0.2: JP6.2 54.77,97 v44,97
  Bottom 0.2: v44,97 43.77,97.23 29.18,97.23 v25.15,93.2
V+  (via drill 0.35)
  Top 0.254: U23.7 50.06,46.1 v49.2,46.1
  Top 0.5: v27.88,16.7 27.8,16.62 27.8,14.85 U22.5
  Top 0.8: C10.+ 54.12,33.06 54.12,39.12 52.12,41.12 52.12,45.09 51.05,46.16 U23.7
  Bottom 0.2: R25.2 48,69.03 | 24.4,52.08 C11.1 | C37.2 46.33,46 | v49.2,46.1 49.05,46.25 49.05,46.36 48.6,46.81 48.6,49.75 48,50.35 R25.2 | 47.85,68.9 R25.2
  Bottom 0.254: v49.2,46.1 50.15,47.05 R43.2
  Bottom 0.3: C11.1 25,52.62 25,53.8 R23.2
  Bottom 0.305: v41.17,23.97 41.17,18.96 D12.C
  Bottom 0.5: v27.88,16.7 U20.4 | C37.2 49.1,46 v49.2,46.1
  other vias: 24.9,22.15 24.9,21.35 24.88,32.42 24.88,31.62 24.9,42.25 24.9,41.45 24.93,52.45 24.93,51.65
  pour Bottom (isolate 0.305, no thermals): 23.73,51.15 23.73,52.95 25.23,52.95 25.23,51.15
  pour Bottom (isolate 0.305, no thermals): 23.7,20.7 23.7,22.78 25.2,22.78 25.2,20.7
  pour Bottom (isolate 0.305, no thermals): 23.68,31.12 23.68,32.92 25.18,32.92 25.18,31.12
  pour Bottom (isolate 0.305, no thermals): 23.7,40.95 23.7,42.75 25.2,42.75 25.2,40.95
  pour Top (isolate 0.5, no thermals): 23.27,52.85 29,52.85 29,7 27,5 25.48,5 23.27,7.2
  pour Top (isolate 0.4, no thermals): 53.42,20.53 53.42,30.7 52.17,31.95 50.67,31.95 49.42,30.7 49.42,28.1 28,28.1 28,23.45 49.42,23.45 49.42,20.58 50.67,19.33 52.23,19.33
V_EXT  (via drill 0.3)
  Top 0.2: X1.13 36.35,103.22 37.1,102.47 37.1,92.92 37.92,92.1 45.9,92.1 v46.17,91.83
  Bottom 0.2: 45.73,73.28 45.5,73.05 45.45,73.05 | 45.73,73.28 46.4,73.95 46.4,91.6 v46.17,91.83 | R27.1 45.45,73.05 | 45.45,73.05 R28.2 45.58,73.28 45.73,73.28
V_GD  (via drill 0.35)
  Top 0.2: R45.2 41.83,57.27
  Top 0.254: U5.1 36.97,49.62 v38.17,49.62 38.08,49.62 | U4.1 v38.15,39.6 38.73,39.03 C7.2 | U3.1 v38.15,29.6 38.2,29.55 C6.2 | U2.1 v38.15,19.6 38.15,19.97 39.52,21.35 C5.2
  Top 0.3: U14.2 40.67,21.08 C5.2 | 38.17,47.9 C8.2 37.98,49.42 v38.17,49.62
  Top 0.4: C39.1 39.58,57.2 36.97,57.2 JP4.1
  Top 0.5: 41.83,57.27 40.5,58.6 | 40.5,58.6 40.5,58.12 C39.1 | 40.5,58.6 D16.C | U25.3 15.75,58.55 v15.9,58.7 16.04,58.84 31.2,58.84 32.19,59.83 35.92,59.83 36.6,59.15 36.57,59.12 JP4.1
  Bottom 0.2: 37.08,49.24 D5.A 37.46,49.62 v38.17,49.62
  Bottom 0.254: v38.15,39.6 38,39.45 37.29,39.45 D4.A | v38.15,29.6 37.85,29.3 D3.A | v38.15,19.6 37.85,19.3 D2.A
  Bottom 0.3: v38.17,49.62 37.39,49.62 37.02,50
  Bottom 0.5: C41.1 15.6,59 v15.9,58.7
  Bottom 1: D2.A 37.17,19.3 37.17,29.3 D3.A 37.14,29.6 37.14,29.61 D4.A 37.02,39.42 37.02,50 37.02,56.8 JP4.1
V_INT  (via drill 0.3)
  Top 0.2: X1.14 37.6,105.02 37.6,93 37.98,92.62 46.84,92.62 v46.93,92.53
  Bottom 0.2: v46.93,92.53 47.05,92.41 47.05,73.97 48,73.03 R26.2 R25.1
V_INT_TMC  (via drill 0.3)
  Top 0.152: v24.55,72.3 24.57,72.3 24.57,67.73 24.3,67.45 24.3,65.3 | U1.20 25.2,81.55 v24.93,81.83 | U18.12 24.3,65.3 | 24.3,65.3 24.3,63.65 24.6,63.35 U18.9 U18.8
  Bottom 0.152: v24.93,81.83 24.43,81.33 24.43,72.58 24.55,72.45 v24.55,72.3
V_INT_TMC_RAW  (via drill 0.3)
  Top 0.2: v24.55,61.15 24.95,61.15 25.95,62.15 25.95,63.95 25.9,64 U18.10
  Bottom 0.2: v24.55,61.15 25.6,60.1 25.6,59 | R23.1 25.6,59 | R24.2 25.6,59
V_MOT_IN  (via drill 0.35)
  Bottom 0.152: C33.2 27.15,12.05
  Bottom 0.2: U20.3 26.02,15.97 26.52,15.47 26.52,14.33 26.78,14.08 U20.6 | v30.43,13.83 30.89,14.29 31.38,14.29 33.94,16.85 37.74,16.85 40.05,19.16 40.05,21.37 40.28,21.6 40.28,27.71 41.4,28.83 41.4,38.62 42.45,39.67 42.45,66.05 R27.2
  Bottom 0.5: v30.43,13.83 30.18,14.08 U20.6 27.53,14.08 27.53,12.43 27.15,12.05
  other vias: 30.43,12.83 32.42,12.83 31.43,12.83 30.43,11.83 31.43,11.83 32.42,11.83 31.43,13.83
  pour Top (isolate 0.4, no thermals): 29.7,14.47 29.7,6.2 30.9,5 34.38,5 34.8,5.42 34.8,8.58 34,9.38 34,12.08 31.6,14.47
  pour Bottom (isolate 0.4, no thermals): 29.7,14.47 29.7,6.2 30.9,5 34.38,5 34.8,5.42 34.8,11.28 31.6,14.47
VCORE  (via drill 0.3)
  Top 0.152: v30.15,71.68 30.15,71.76 30.42,72.02 U1.45 | U1.15 27.04,83.55 26.87,83.72 v26.87,84.9 | v35.48,78.1 35.23,78.35 U1.63
  Bottom 0.152: C3.2 26.87,84.38 v26.87,84.9 | v35.48,78.1 35.48,78.67 C4.2
  Bottom 0.2: v30.15,71.68 30.15,71.75 C1.2 30.93,72.78 30.3,73.4 30.3,75.85 29.4,76.75 27.43,76.75 26.77,77.4 26.77,83.3 27.07,83.6 C3.2 30.77,80.47 34.08,80.47 35.02,79.53 C4.2
VREF_A_RAW  (via drill 0.35)
  Top 0.2: U6.6 11.87,47.47 v12,47.6
  Bottom 0.2: v12,47.6 12.15,47.75 C43.1 12.65,48.55 13.2,49.1 13.2,50.9 13.1,51 JP14.1
VREF_C_RAW  (via drill 0.35)
  Top 0.2: v11.55,29.11 11.72,28.94 11.72,27.62 U7.6
  Bottom 0.2: C42.1 11.5,32.23 10.7,31.43 10.7,29.77 11.36,29.11 v11.55,29.11
  Bottom 0.25: C42.1 11.5,37 JP13.1

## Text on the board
tPlace: E-Stop | EN | GND | 5V | 3V3 | P | N | 2.5V -> N / (Single ended) | V | AENC | RX | U|X | TX | W|Y | GND | 5V | 7 | 6 | UART (3V3) | 3V3 | 2V5 / N Offset | GND | 4 | 5 | 5V | R | GPIO | 3 | 2 | Z | AGPI_A | Z | 0 | B | H | ENC | 1 | ENO | L | B | ENC2 (3V3) | A | TMC4671 | A | PWM | GND | STP | 5V | DIR | WY | PWR | V | HALL | UX | GND | + | 5V | 10V | A | MOTOR | B | C | D | 3 phase / ABC = UVW | MOTOR / A|B|C|D | GND | PB+ | VM | PB- | Power | SUPPLY / 1:GND / 2:PB+ / 3:VM + / 4:PB-
bPlace: 5V | E-Stop | 16 | 2 | 1 | GND | 5V | RST | 3V3 | MOSI | MISO | CS1 | SCK | CS2 | CS3 | FLAG | BRK | V_EXT | V_INT | NC | ENABLE | EN | GND | P | N | V | RX | UART | U | TX | Cos | 1 | 2 | 3 | AENC | GND | W | Sin | N/CM | 2V5 | 3V3 | 5V | N Offset | SPI ADDR | 5V | GND | ENC2 (3V3) | Z | R | 5V | B | H | Z | A | L | B | PWM | A | ENCODER | VEXT | VINT | STP | GND | DIR | 5V | WY | V | HALL | BR_TH | 2V5-REF / Sense | UX | GND | 5V | V_GD / (10V) | STEPPER: AB(A) CD(B) | 3 PHASE: ABC(UVW) | DC: AB | Open FFBoard - TMC4671 Motor driver | A | MOTOR | B | TMP | C | GIT version / V1.3.3 - YR 2023 / ACS724 30 (66mV/A) | D | Supply: / PSU (protected): VM (+) and GND (-) / ALWAYS connect braking resistor / between PB+ and PB- | R | VM | GND | PB+ | PB- | - | + | Power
